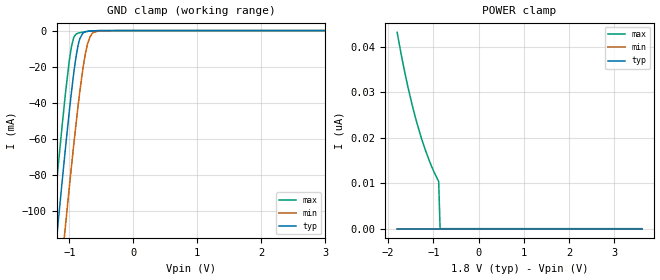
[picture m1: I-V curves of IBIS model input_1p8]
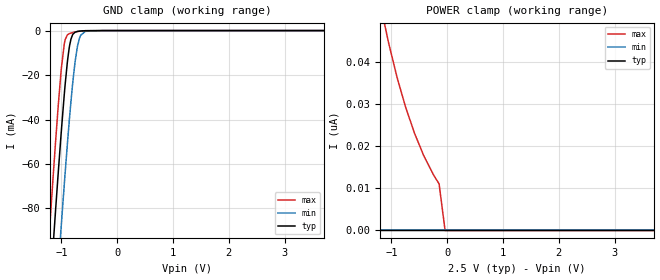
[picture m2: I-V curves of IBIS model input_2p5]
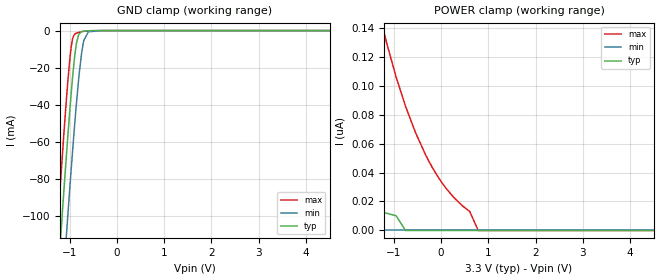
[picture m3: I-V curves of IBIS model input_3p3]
|Texas Instruments Incorporated
| Single Power Supply Single Buffer GATE with 3-State Output CMOS Logic
| Level Shifter
| Marketing part#   Digital Voltage Range   Package-type   #pins
| SN74LV1T125DBVR   1.6V-5.5V   SOT-23   5
| SN74LV1T125DCKR   1.6V-5.5V   SC70   5
[IBIS Ver]   4.1
[File name]   sn74lv1t125.ibs
[File Rev]   2.0
[Date]   12/31/2013
[Source]
| Texas Instruments Incorporated.
| Analog-eLab Design Center, HPA
| 12500 TI Blvd
| Dallas, TX -75243
[Notes]   Revision History:
| Rev 1.0: 11/08/2013
| - Initial model based on 5V parent device AHCT1G125.
| Rev 2.0: 12/31/2013
| - All new models including 5V.
| - Model generated from simulations in TISPICE
| - Model matched to SPICE simulation
| - C_comp although listed in numerical order of value are
|   obtained from varying PVT conditions. For PVT conditions for
|   each specific value refer the buffer description under
|   respective [Model]. IBIS model user is responsible for using
|   appropriate C_comp to simulate for Signal Integrity.
[Disclaimer]
| This model is designed as an aid for customers of Texas Instruments.
| TI and its licensors and suppliers make no warranties, either expressed
| or implied, with respect to this  model, including the warranties of
| merchantability or fitness for a particular purpose. The model is
| provided solely on an "as is" basis. The entire risk as to its quality
| and performance is with the customer.
[Copyright]
(C) Copyright 2013 Texas Instruments Incorporated.All rights reserved.
|   SN74LV1T125DBV
[Component]   SN74LV1T125DBV
[Manufacturer]   TI
[Package]   |5 SOT-23  -  DBV package
|   typ   min   max
R_pkg   0.06209   0.05045   0.07001
L_pkg   1.83153nH   1.49378nH   2.04843nH
C_pkg   0.26256pF   0.24997pF   0.27952pF
[Pin]  signal_name   model_name   R_pin   L_pin   C_pin
1   _OE   INPUT   0.07001   2.04843nH  0.27952pF
2   A   INPUT   0.05045   1.49378nH  0.25820pF
3   GND   GND   0.06850   2.45772nH  0.39635pF
4   Y   OUTPUT   0.06582   1.95239nH  0.24997pF
5   VCC   POWER   0.06589   1.95370nH  0.25029pF
|   SN74LV1T125DCK
[Component]   SN74LV1T125DCK
[Manufacturer]   TI
[Package]   |5 SC70   -  DCK package
|   typ   min   max
R_pkg   0.04747   0.04577   0.04900
L_pkg   1.58367nH   1.46085nH   1.66427nH
C_pkg   0.23613pF   0.22997pF   0.24076pF
[Pin]  signal_name   model_name   R_pin   L_pin   C_pin
1   _OE   INPUT   0.04900   1.62590nH  0.24076pF
2   A   INPUT   0.04577   1.46085nH  0.23766pF
3   GND   GND   0.04635   1.67071nH  0.26247pF
4   Y   OUTPUT   0.04763   1.66427nH  0.22997pF
5   VCC   POWER   0.04778   1.66679nH  0.23019pF
|   Model Selectors
[Model Selector] INPUT
input_1p8   1.8V  digital input
input_2p5   2.5V  digital input
input_3p3   3.3V  digital input
input_5p0   5.0V  digital input
[Model Selector] OUTPUT
output_1p8   1.8V  digital 3-state
output_2p5   2.5V  digital 3-state
output_3p3   3.3V  digital 3-state
output_5p0   5.0V  digital 3-state
| Models and submodels in the file (8): input_1p8 (Input), input_2p5 (Input), input_3p3 (Input), input_5p0 (Input), output_1p8 (3-state), output_2p5 (3-state), output_3p3 (3-state), output_5p0 (3-state)
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|   input_1p8 Model
[Model]   input_1p8
Model_type   Input
Vinl = 0.57
Vinh = 0.95
|   typ   min   max
|   (nom PVT)   (fast PVT)   (slow PVT)
C_comp   6.973e-13   6.927e-13   7.020e-13
[Model spec]
|subparameter
Vinl   0.57   0.57   0.57
Vinh   0.95   0.95   0.99
| Where nom  PVT is Nominal Process, 1.8V, 40C
|   Fast PVT is Strong Process,  1.98V, -40C
|   Slow PVT is Weak Process,   1.62V, 140C
[Voltage Range]   1.8   1.62   1.98
|Junction Temperature
[Temperature Range]   40   140   -40
[Power Clamp Reference]   1.8   1.62   1.98
[GND Clamp Reference]   0   0   0
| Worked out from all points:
|   GND clamp passes 1 mA (typ) near -0.77 V on its own axis
[GND Clamp]
|   Voltage   I(typ)   I(min)   I(max)
-1.8V     -349mA     -390mA     -320.7mA
-1.4V     -191.8mA   -234.7mA   -161.5mA
-1.2V     -115.7mA   -159.1mA   -84.63mA
-1.165V   -102.5mA   -145.9mA   -71.47mA
-1.071V   -68.72mA   -111.8mA   -38.32mA
-968.4mV  -34.53mA   -75.73mA   -9.255mA
-887.4mV  -12.81mA   -49.13mA   -1.824mA
-833.4mV  -4.24mA    -33.01mA   -1.152mA
-750.2mV  -670.7uA   -12.99mA   -614.3uA
-680.6mV  -250.8uA   -3.714mA   -303.4uA
-623.9mV  -121.5uA   -1.06mA    -143.4uA
3.6V      0A         0A         0A
[POWER Clamp]
|   Voltage   I(typ)   I(min)   I(max)
-1.8V     0A         0A         43.21nA
-1.675V   0A         0A         36.55nA
-1.588V   0A         0A         32.38nA
-1.457V   0A         0A         26.8nA
-1.366V   0A         0A         23.36nA
-1.251V   0A         0A         19.51nA
-1.085V   0A         0A         14.84nA
-984.2mV  0A         0A         12.45nA
-883.1mV  0A         0A         10.37nA
-851.4mV  0A         0A         0A
3.6V      0A         0A         0A
|   input_2p5 Model
[Model]   input_2p5
Model_type   Input
Vinl = 0.75
Vinh = 1.145
|   typ   min   max
|   (nom PVT)   (fast PVT)   (slow PVT)
C_comp   6.859e-13   6.814e-13   6.904e-13
[Model spec]
|subparameter
Vinl   0.75   0.75   0.75
Vinh   1.145   1.145   1.22
| Where nom  PVT is Nominal Process, 2.5V, 40C
|   Fast PVT is Strong Process,  2.75V, -40C
|   Slow PVT is Weak Process,   2.25V, 140C
[Voltage Range]   2.5   2.25   2.75
|Junction Temperature
[Temperature Range]   40   140   -40
[Power Clamp Reference]   2.5   2.25   2.75
[GND Clamp Reference]   0   0   0
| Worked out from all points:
|   GND clamp passes 1 mA (typ) near -0.77 V on its own axis
[GND Clamp]
|   Voltage   I(typ)   I(min)   I(max)
-2.5V     -629.8mA   -667.3mA   -604.3mA
-1.232V   -127.8mA   -171.2mA   -96.85mA
-1.145V   -95.5mA    -138.9mA   -64.49mA
-1.105V   -80.81mA   -124.1mA   -50mA
-1.008V   -47.03mA   -89.23mA   -18.62mA
-943mV    -26.96mA   -67.16mA   -5.2mA
-862.5mV  -8.087mA   -41.49mA   -1.429mA
-792.3mV  -1.573mA   -22.16mA   -860.5uA
-713.5mV  -383.8uA   -7.11mA    -434.7uA
-654.8mV  -181.4uA   -2.119mA   -220.4uA
-571.7mV  -57.55uA   -335.5uA   -61.53uA
5V        0A         0A         0A
[POWER Clamp]
|   Voltage   I(typ)   I(min)   I(max)
-2.5V     17.64nA    0A         203.4nA
-1.738V   10.07nA    0A         99.15nA
-1.675V   0A         0A         92.8nA
-1.185V   0A         0A         52.7nA
-1.051V   0A         0A         44.4nA
-890mV    0A         0A         35.79nA
-748.2mV  0A         0A         29.29nA
-587.5mV  0A         0A         23.05nA
-423.8mV  0A         0A         17.78nA
-146mV    0A         0A         11.01nA
-38.75mV  0A         0A         0A
5V        0A         0A         0A
|   input_3p3 Model
[Model]   input_3p3
Model_type   Input
Vinl = 0.8
Vinh = 1.37
|   typ   min   max
|   (nom PVT)   (fast PVT)   (slow PVT)
C_comp   6.770e-13   6.726e-13   6.814e-13
[Model spec]
|subparameter
Vinl   0.8   0.8   0.8
Vinh   1.37   1.37   1.47
| Where nom  PVT is Nominal Process, 3.3V, 40C
|   Fast PVT is Strong Process,  3.6V, -40C
|   Slow PVT is Weak Process,   3V, 140C
[Voltage Range]   3.3   3   3.6
|Junction Temperature
[Temperature Range]   40   140   -40
[Power Clamp Reference]   3.3   3   3.6
[GND Clamp Reference]   0   0   0
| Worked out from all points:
|   GND clamp passes 1 mA (typ) near -0.76 V on its own axis
[GND Clamp]
|   Voltage   I(typ)   I(min)   I(max)
-3.3V     -954.2mA   -987.6mA   -931.2mA
-1.647V   -288.4mA   -330.2mA   -259.4mA
-1.252V   -135mA     -178.4mA   -104.1mA
-1.226V   -125.5mA   -168.9mA   -94.54mA
-1.126V   -88.25mA   -131.6mA   -57.31mA
-1.065V   -66.62mA   -109.6mA   -36.32mA
-966.9mV  -34.07mA   -75.22mA   -8.966mA
-861mV    -7.844mA   -41.04mA   -1.412mA
-795.3mV  -1.688mA   -22.9mA    -880.2uA
-712.8mV  -380.1uA   -7.022mA   -431.6uA
-603mV    -91.15uA   -664.8uA   -104.1uA
6.6V      0A         0A         0A
[POWER Clamp]
|   Voltage   I(typ)   I(min)   I(max)
-3.3V     46.68nA    0A         641.2nA
-2.436V   28.44nA    0A         371.7nA
-1.345V   13.71nA    0A         155.4nA
-1.171V   12.05nA    0A         132nA
-952.8mV  10.19nA    0A         106.1nA
-751.2mV  0A         0A         85.68nA
-542.4mV  0A         0A         67.68nA
-330mV    0A         0A         52.37nA
112.8mV   0A         0A         28.82nA
607.2mV   0A         0A         13.09nA
786mV     0A         0A         0A
6.6V      0A         0A         0A
